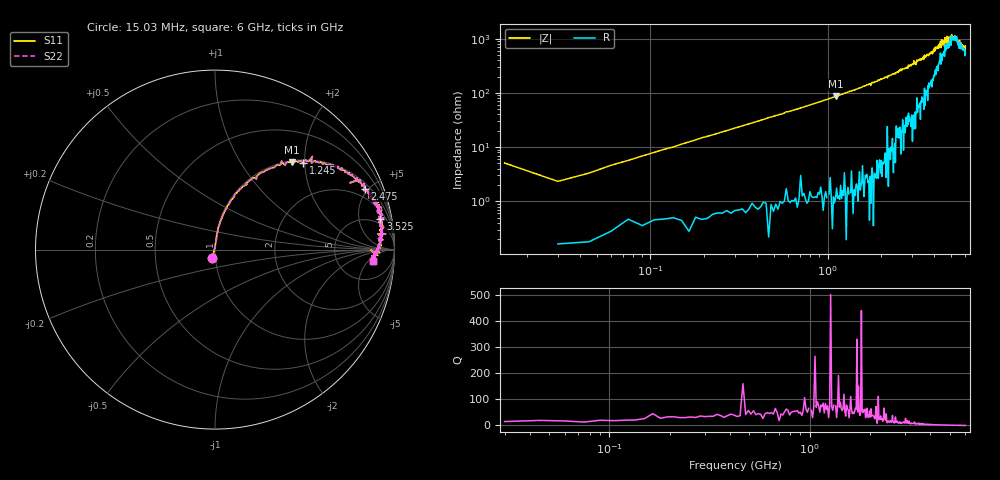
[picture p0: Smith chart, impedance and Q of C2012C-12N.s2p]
!	Network	Analyzer	HP8753E.07.74:	Oct	30	2002	Serial	No.	JP38451487
!	Hewlett-Packard
!	7	Sep	2009	10:44:24
!	Frequency	S11	S21	S12	S22
#	HZ	S	RI	R	50
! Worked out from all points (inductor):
!   400 points, 15.03 MHz to 6 GHz, reference 50 ohm
!   read as one part in series: L = 12 nH near 45.03 MHz
!   highest Q = 74.8 at 1.11 GHz (marker M1), where L = 12.4 nH
!   self-resonance near 5.334 GHz
!   S11 on the Smith chart (normalised r, x): 15.03 MHz: 0.97, -0.09; 1.245 GHz: 1.07, +1.96; 2.475 GHz: 1.33, +4.74; 3.525 GHz: 3, +10; 6 GHz: 12, -7
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1.502992e7  -0.0153 -0.0488  1.02 0.0488  1.02 0.0488  -0.0153 -0.0488
3.002985e7  0.00235 0.0232  0.998 -0.0232  0.998 -0.0232  0.00235 0.0232
6.00297e7  0.00485 0.0459  0.995 -0.0459  0.995 -0.0459  0.00485 0.0459
1.200294e8  0.0127 0.0897  0.987 -0.0897  0.987 -0.0897  0.0127 0.0897
2.850286e8  0.0488 0.202  0.951 -0.202  0.951 -0.202  0.0488 0.202
5.850271e8  0.177 0.363  0.823 -0.363  0.823 -0.363  0.177 0.363
1.020025e9  0.381 0.477  0.619 -0.477  0.619 -0.477  0.381 0.477
1.110024e9  0.427 0.488  0.573 -0.488  0.573 -0.488  0.427 0.488
1.245024e9  0.491 0.483  0.509 -0.483  0.509 -0.483  0.491 0.483
2.01002e9  0.754 0.415  0.246 -0.415  0.246 -0.415  0.754 0.415
2.475018e9  0.833 0.34  0.167 -0.34  0.167 -0.34  0.833 0.34
3.015015e9  0.911 0.266  0.0886 -0.266  0.0886 -0.266  0.911 0.266
3.525012e9  0.921 0.171  0.0787 -0.171  0.0787 -0.171  0.921 0.171
4.00501e9  0.938 0.129  0.0618 -0.129  0.0618 -0.129  0.938 0.129
4.575007e9  0.907 0.0872  0.0927 -0.0872  0.0927 -0.0872  0.907 0.0872
4.605007e9  0.931 0.0563  0.0695 -0.0563  0.0695 -0.0563  0.931 0.0563
5.010005e9  0.917 0.0311  0.0826 -0.0311  0.0826 -0.0311  0.917 0.0311
5.355003e9  0.918 -0.0183  0.0821 0.0183  0.0821 0.0183  0.918 -0.0183
5.535002e9  0.869 -0.00217  0.131 0.00217  0.131 0.00217  0.869 -0.00217
5.565002e9  0.908 -0.0334  0.092 0.0334  0.092 0.0334  0.908 -0.0334
5.595002e9  0.879 -0.0101  0.121 0.0101  0.121 0.0101  0.879 -0.0101
6e9  0.882 -0.0645  0.118 0.0645  0.118 0.0645  0.882 -0.0645
